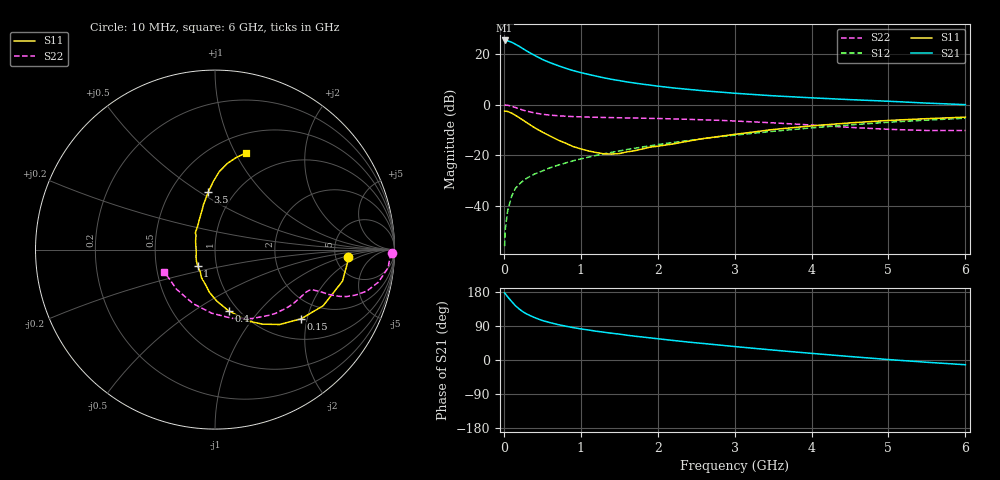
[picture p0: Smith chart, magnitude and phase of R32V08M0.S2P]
! SIEMENS Small Signal Semiconductors
! BFR181
! Si NPN RF Bipolar Junction Transistor in SOT23
! VCE = 2 V  IC = 8 mA
! Common Emitter S-Parameters:  May  1996
# GHz  S  MA  R  50
!  f  S11  S21  S12  S22
! GHz  MAG  ANG  MAG  ANG  MAG  ANG  MAG  ANG
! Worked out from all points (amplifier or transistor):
!   36 points, 10 MHz to 6 GHz, reference 50 ohm
!   highest |S21| = 25.3 dB at 10 MHz (marker M1)
!   |S21| within 3 dB of that: start of sweep to 235.5 MHz
!   unconditionally stable (mu >= 1): 789.2 MHz to 2.742 GHz
!   at 250 MHz: K = 0.57, MSG = 26.1 dB, |S12| = -30.1 dB
!   at 1.4 GHz: K = 1.08, MAG = 12.7 dB, |S12| = -18.9 dB
!   at 6 GHz: K = 0.86, MSG = 2.7 dB, |S12| = -5.4 dB
!   S11 on the Smith chart (normalised r, x): 10 MHz: 6.55, -1.17; 150 MHz: 1.48, -1.84; 400 MHz: 0.90, -0.70; 1 GHz: 0.81, -0.15; 3.5 GHz: 0.76, +0.54; 6 GHz: 0.70, +1.10
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0.01  0.7425 -3.1  18.46 177.2  0.0016 95.6  0.9836 -1.1
0.02  0.7419 -5.6  18.3 174.4  0.0036 84.4  0.9765 -2.4
0.05  0.7316 -13.9  18.18 166.7  0.008 82.9  0.9696 -6.0
0.1  0.6791 -27.4  17.09 154.7  0.0153 76.1  0.9281 -11.3
0.15  0.6155 -38.8  15.57 143.3  0.0221 72.2  0.8764 -15.3
0.2  0.5506 -49.3  14.14 134.5  0.0267 70.3  0.824 -17.9
0.25  0.4918 -57.6  12.65 127.1  0.0313 67.5  0.7765 -19.7
0.3  0.4382 -65.1  11.36 121.1  0.0353 66.9  0.7402 -20.6
0.4  0.3491 -77.5  9.356 111.9  0.0427 65.7  0.6834 -21.5
0.5  0.2871 -88.0  7.806 104.2  0.0489 66.2  0.6441 -21.7
0.6  0.2399 -97.4  6.733 98.7  0.0565 66.6  0.6189 -21.9
0.7  0.2011 -105.5  5.914 93.7  0.0633 67.2  0.6026 -22.2
0.8  0.1737 -115.7  5.233 89.4  0.0701 67.2  0.5888 -22.4
1  0.1336 -136.2  4.283 82.1  0.0845 68.2  0.5727 -23.3
1.1  0.1215 -148.3  3.947 79.2  0.0917 68.4  0.5661 -24.1
1.3  0.1066 -169.0  3.377 73.4  0.1068 68.2  0.5566 -25.7
1.6  0.1164 158.5  2.805 65.4  0.1295 67.6  0.5456 -29.0
2.2  0.1669 124.7  2.135 51.6  0.1785 64.9  0.522 -37.0
3.5  0.322 96.8  1.491 26.2  0.2967 54.7  0.436 -61.8
4.5  0.435 86.9  1.253 9.2  0.3975 43.6  0.3547 -93.0
5.5  0.5274 76.9  1.069 -6.0  0.4939 30.4  0.3078 -134.0
6  0.5648 72.2  0.997 -12.5  0.5377 23.2  0.3079 -156.2
